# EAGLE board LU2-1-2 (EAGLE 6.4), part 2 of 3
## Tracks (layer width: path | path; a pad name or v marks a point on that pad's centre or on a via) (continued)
N$65 (continued)
  Top 0.305: IC5.13 44.45,78.74 43.18,77.47 43.18,73.66 44.45,72.39 IC4.13 44.45,67.31 43.18,66.04 43.18,62.23 40.64,59.69 40.64,55.88 38.42,53.66 38.42,40.32 37.47,39.37 IC33.15
N$66
  Top 0.305: IC5.11 49.53,78.74 48.26,77.47 48.26,73.66 49.53,72.39 IC4.11 49.53,66.67 48.26,65.41 48.26,56.52 46.35,54.61 41.91,54.61 39.69,52.32 39.69,33.02 38.42,31.75 IC33.12
N$67
  Top 0.305: IC4.8 44.45,77.47 45.72,78.74 45.72,83.19 44.45,84.45 IC5.8
  Route3 0.305: IC33.9 43.81,31.75 45.09,33.02 45.09,53.98 45.72,54.61 45.72,71.75 44.45,73.03 IC4.8
N$68
  Top 0.305: IC4.6 39.37,77.47 40.64,78.74 40.64,83.19 39.37,84.45 IC5.6
  Route3 0.305: IC33.6 44.45,40.64 44.45,53.98 43.18,55.24 43.18,69.22 39.37,73.03 IC4.6
N$69
  Top 0.305: IC4.4 34.29,77.47 35.56,78.74 35.56,83.19 34.29,84.45 IC5.4
  Route3 0.305: IC4.4 34.29,72.39 35.56,71.12 35.56,62.23 38.1,59.69 38.1,45.09 41.27,41.91 IC33.5
N$70
  Top 0.305: IC4.2 29.21,77.47 30.48,78.74 30.48,84.45 29.21,85.72 IC5.2
  Route3 0.305: IC4.2 31.11,78.11 34.92,78.11 35.56,77.47 35.56,73.66 38.1,71.12 38.1,62.23 40.64,59.69 40.64,50.16 41.27,49.53 IC33.2
N$71  (via drill 0.6)
  Top 0.305: JP8.4 96.52,41.91 94.61,43.81 94.61,72.07 v94.3,72.39
  Route2 0.305: v94.3,72.39 118.75,72.39 120.65,70.48 IC7.12
  Bottom 0.305: JP7.4 JP8.4
N$75
  Top 0.305: LED14.K R26.2
N$77  (via drill 0.6)
  Top 0.305: JP8.5 96.52,44.45 95.25,45.72 95.25,73.03 v94.61,73.66
  Bottom 0.305: JP8.5 JP7.5 | IC7.9 120.65,74.3 119.38,73.03 95.89,73.03 95.25,73.66 v94.61,73.66
N$78
  Top 0.305: SV1.6 180.97,45.09 180.97,38.73 180.34,38.1 IC35.7
  Bottom 0.305: SV1.6 RN9.4 | IC20.13 162.56,35.56 163.83,36.83 175.26,36.83 176.53,38.1 IC35.7
N$79  (via drill 0.6)
  Top 0.305: JP8.6 96.52,46.99 95.89,47.62 95.89,74.3 94.93,75.25 v94.3,75.25
  Bottom 0.305: JP7.6 JP8.6 | IC7.7 115.57,74.3 114.94,73.66 96.52,73.66 94.93,75.25 v94.3,75.25
N$84  (via drill 0.6)
  Top 0.305: JP8.7 96.52,50.8 96.52,74.93 v95.25,76.2
  Bottom 0.305: JP8.7 JP7.7 | IC7.5 110.49,74.93 109.86,74.3 97.16,74.3 v95.25,76.2
N$85  (via drill 0.6)
  Top 0.305: JP8.8 97.79,53.34 97.16,53.98 97.16,75.88 v96.84,76.2
  Bottom 0.305: JP7.8 JP8.8 | IC7.3 105.41,75.56 104.78,74.93 98.11,74.93 v96.84,76.2
N$86
  Top 0.305: U6.A0 99.06,22.23 97.79,23.5 97.79,24.77 98.42,25.4 102.87,25.4 104.46,26.99 104.46,46.67 104.14,46.99 IC8.18
N$87
  Top 0.305: U6.A1 96.52,22.23 95.25,23.5 95.25,25.4 95.89,26.04 102.23,26.04 103.82,27.62 103.82,41.59 103.5,41.91 IC8.16
N$88
  Top 0.305: U6.A2 93.98,22.23 92.71,23.5 92.71,25.4 93.98,26.67 101.6,26.67 103.19,28.26 103.19,36.51 102.87,36.83 IC8.14
N$89
  Top 0.305: U6.A3 91.44,22.23 90.17,23.5 90.17,25.4 92.08,27.3 99.06,27.3 100.33,28.57 100.33,30.48 IC8.12
N$90
  Top 0.305: RN5.9 107.95,121.28 109.22,120.02 109.22,116.84 U9.K0
N$91
  Top 0.305: RN5.8 105.41,121.28 106.68,120.02 106.68,117.47 105.41,116.2 U9.K1
N$92
  Route2 0.305: IC8.9 106.68,31.75 102.87,27.94 92.08,27.94 90.17,26.04 90.17,22.86 88.9,21.59 U6.A4
N$93  (via drill 0.6)
  Top 0.305: IC8.7 108.58,36.83 107.95,36.2 107.95,25.4 107.95,24.77 107.95,20.95 v107.31,20.32
  Bottom 0.305: U6.A5 87.63,21.59 100.33,21.59 101.6,20.32 v107.31,20.32
N$94  (via drill 0.6)
  Top 0.305: IC8.5 108.58,41.91 107.31,40.64 107.31,22.86 v106.68,22.23
  Bottom 0.305: U6.A6 83.82,20.95 85.09,22.23 v106.68,22.23
N$95  (via drill 0.6)
  Top 0.305: IC8.3 108.58,46.99 107.63,46.04 107.63,43.5 106.68,42.55 106.68,24.13 v106.05,23.5
  Bottom 0.305: U6.A7 81.28,22.23 81.92,22.86 105.41,22.86 v106.05,23.5
N$96
  Top 0.305: RN15.2 99.06,23.5 100.33,22.23 100.33,19.68 99.06,18.41 U6.K0
N$97
  Top 0.305: RN15.3 96.52,23.5 97.79,22.23 97.79,19.68 96.52,18.41 U6.K1
N$98
  Top 0.305: RN15.4 93.98,23.5 95.25,22.23 95.25,19.68 93.98,18.41 U6.K2
N$99
  Top 0.305: RN15.5 91.44,23.5 92.71,22.23 92.71,19.68 91.44,18.41 U6.K3
N$100
  Top 0.305: RN15.6 88.9,23.5 90.17,22.23 90.17,19.68 88.9,18.41 U6.K4
N$101
  Top 0.305: RN5.7 102.87,121.28 104.14,120.02 104.14,117.47 102.87,116.2 U9.K2
N$102  (via drill 0.6)
  Top 0.305: v160.02,113.03 160.02,93.98 v158.75,92.71
  Route2 0.305: IC26.2 64.77,88.9 66.04,90.17 95.89,90.17 97.79,92.08 158.12,92.08 v158.75,92.71
  Route3 0.305: IC26.2 64.77,86.36 63.5,85.09 63.5,27.3 62.23,26.04 62.23,10.16 60.96,8.89 60.96,5.08 59.69,3.81 54.61,3.81 SW11.2
  Bottom 0.305: IC24.2 184.15,114.94 183.51,114.3 161.29,114.3 v160.02,113.03
N$103
  Top 0.305: R25.2 LED13.K
N$104
  Top 0.305: LED12.K R24.2
N$105
  Top 0.305: RN15.7 86.36,23.5 87.63,22.23 87.63,19.68 86.36,18.41 U6.K5
N$106
  Top 0.305: U6.K6 83.82,18.41 85.09,19.68 85.09,22.23 83.82,23.5 RN15.8
N$107
  Top 0.305: RN15.9 81.28,23.5 82.55,22.23 82.55,19.68 81.28,18.41 U6.K7
N$108  (via drill 0.6)
  Top 0.305: v106.68,44.45 106.68,50.16 102.87,53.98 IC6.19 102.87,59.05 106.68,62.87 106.68,66.04 107.95,67.31 IC7.17
  Bottom 0.305: v106.68,44.45 IC8.17
N$109  (via drill 0.6)
  Top 0.305: IC7.15 113.03,66.67 111.76,65.41 111.76,61.59 110.49,60.33 IC6.16 110.49,55.88 111.12,55.24 111.12,41.27 v110.49,40.64
  Bottom 0.305: v110.49,40.64 106.05,40.64 104.78,39.37 IC8.15
N$110  (via drill 0.6)
  Top 0.305: IC7.13 118.11,67.31 116.84,66.04 116.84,63.5 113.03,59.69 IC6.15 113.03,55.88 114.3,54.61 114.3,38.73 113.67,38.1 112.39,38.1 111.76,37.47 111.76,36.83 v110.49,35.56
  Bottom 0.305: v110.49,35.56 106.68,35.56 105.41,34.29 IC8.13
N$111  (via drill 0.6)
  Top 0.305: IC7.11 123.19,67.31 121.92,66.04 121.92,61.59 120.65,60.33 IC6.12 120.65,55.88 118.11,53.34 118.11,36.2 117.47,35.56 v117.47,31.11
  Bottom 0.305: IC8.11 102.87,29.21 104.14,30.48 116.84,30.48 v117.47,31.11
N$112
  Top 0.305: IC7.8 118.11,73.03 119.38,71.75 119.38,67.31 120.65,66.04 IC6.9 120.65,61.59 119.38,60.33 119.38,55.88 117.47,53.98 117.47,36.83 116.2,35.56 112.39,35.56 111.12,34.29 IC8.8
N$113
  Top 0.305: IC7.6 113.03,73.03 114.3,71.75 114.3,66.67 113.03,65.41 IC6.6 113.03,61.59 111.76,60.33 111.76,40.01 111.12,39.37 IC8.6
N$114
  Top 0.305: IC7.4 107.95,74.3 111.76,70.48 111.76,67.31 110.49,66.04 IC6.5 110.49,61.59 109.22,60.33 109.22,55.88 110.49,54.61 110.49,45.72 IC8.4
N$115
  Top 0.305: IC6.2 102.87,66.04 104.14,67.31 104.14,69.85 | 104.14,69.85 104.14,71.75 102.87,73.03 IC7.2 | IC8.2 108.58,49.53 106.68,51.44 106.68,60.33 109.22,62.87 109.22,69.22 108.58,69.85 104.14,69.85
N$116  (via drill 0.6)
  Top 0.305: JP6.1 88.27,34.29 86.36,36.2 86.36,55.88 87,56.52 87,62.23 v87.63,62.87
  Bottom 0.305: RN22.2 JP5.1 JP6.1 | v87.63,62.87 89.53,62.87 90.17,63.5 104.78,63.5 105.41,64.14 IC6.3
N$117
  Top 0.305: LED11.K R23.2
N$118  (via drill 0.6)
  Top 0.305: IC24.12 201.93,104.78 202.56,104.14 202.56,84.45 208.91,78.11 208.91,44.13 210.19,42.86 210.19,16.51 208.28,14.61 v208.28,9.84
  Route2 0.305: LED14.A 144.78,11.43 151.76,11.43 152.4,12.06 157.48,12.06 158.12,11.43 165.74,11.43 166.37,12.06 202.56,12.06 205.1,9.53 207.96,9.53 v208.28,9.84
N$119  (via drill 0.6)
  Top 0.305: IC24.14 198.75,106.05 198.75,85.72 207.65,76.83 207.65,42.23 208.91,40.96 208.91,17.78 207.01,15.88 207.01,12.06 v206.38,11.43
  Route2 0.305: LED13.A 114.3,13.97 168.91,13.97 169.54,13.34 203.2,13.34 205.1,11.43 v206.38,11.43
N$120  (via drill 0.6)
  Top 0.305: JP6.2 88.27,36.83 87,38.1 87,53.34 87.63,53.98 89.53,53.98 90.81,55.24 90.81,59.69 90.17,60.33 v90.17,61.59
  Bottom 0.305: RN22.3 JP5.2 JP6.2 | v90.17,61.59 90.17,62.23 90.81,62.87 107.31,62.87 107.95,63.5 IC6.4
N$121  (via drill 0.6)
  Top 0.305: IC24.16 195.58,104.14 195.58,87.63 207.01,76.2 207.01,41.27 208.28,40.01 208.28,18.41 205.74,15.88 v205.74,13.97
  Route2 0.305: LED12.A 85.09,15.24 169.54,15.24 170.18,14.61 205.1,14.61 v205.74,13.97
N$122  (via drill 0.6)
  Top 0.305: JP6.3 87.63,40.64 87.63,52.7 88.27,53.34 90.17,53.34 91.44,54.61 v91.44,60.96
  Bottom 0.305: RN22.4 JP5.3 JP6.3 | v91.44,60.96 92.08,61.59 113.03,61.59 115.57,64.14 IC6.7
N$123  (via drill 0.6)
  Top 0.305: v116.2,53.98 116.84,54.61 116.84,60.33 118.11,61.59 IC6.8
  Bottom 0.305: RN22.5 JP5.4 JP6.4 89.53,41.91 90.81,43.18 99.06,43.18 100.33,44.45 100.33,52.7 100.97,53.34 109.86,53.34 110.49,53.98 v116.2,53.98
N$124
  Bottom 0.305: RN22.6 JP5.5 JP6.5 90.17,45.72 98.42,45.72 99.69,46.99 99.69,53.34 100.33,53.98 109.22,53.98 110.49,55.24 117.47,55.24 118.11,55.88 IC6.13
N$125
  Bottom 0.305: RN22.7 JP5.6 JP6.6 90.17,48.26 98.42,48.26 99.06,48.9 99.06,53.98 99.69,54.61 108.58,54.61 109.86,55.88 114.94,55.88 115.57,56.52 IC6.14
N$126
  Bottom 0.305: RN22.8 JP5.7 | 83.19,49.53 JP5.7 | JP5.7 JP6.7 89.53,49.53 90.17,50.16 90.17,53.98 91.44,55.24 107.31,55.24 107.95,55.88 IC6.17
N$127
  Bottom 0.305: RN22.9 JP5.8 JP6.8 88.9,53.98 90.81,55.88 104.78,55.88 105.41,56.52 IC6.18
N$128  (via drill 0.6)
  Route2 0.305: v134.94,70.17 135.25,70.48 141.6,70.48 142.24,69.85 IC10.18
  Route3 0.305: JP12.1 129.54,34.29 130.81,35.56 130.81,52.7 132.72,54.61 132.72,67.94 v134.94,70.17
  Bottom 0.305: JP11.1 JP12.1
N$129  (via drill 0.6)
  Route2 0.305: IC10.16 147.32,69.85 146.05,71.12 133.99,71.12 v133.35,70.48
  Route3 0.305: JP12.2 128.91,36.83 130.18,38.1 130.18,53.02 132.08,54.93 132.08,69.22 v133.35,70.48
  Bottom 0.305: JP11.2 JP12.2
N$130  (via drill 0.6)
  Route2 0.305: IC10.14 152.4,69.85 150.5,71.75 v132.4,71.75
  Route3 0.305: JP12.3 128.91,39.37 129.54,40.01 129.54,53.34 131.44,55.24 131.44,70.8 v132.4,71.75
  Bottom 0.305: JP11.3 JP12.3
N$131  (via drill 0.6)
  Route2 0.305: IC10.12 157.48,69.85 154.31,73.66 v132.72,73.66
  Route3 0.305: JP11.4 123.19,41.91 125.09,43.81 125.09,53.02 125.41,53.34 128.59,53.34 130.81,55.56 130.81,71.75 v132.72,73.66
  Bottom 0.305: JP11.4 JP12.4
N$132  (via drill 0.6)
  Route2 0.305: IC10.9 156.21,74.93 133.35,74.93 v132.72,75.56
  Route3 0.305: JP11.5 123.19,44.45 124.46,45.72 124.46,53.34 125.09,53.98 128.27,53.98 130.18,55.88 130.18,72.71 132.72,75.25 v132.72,75.56
  Bottom 0.305: JP11.5 JP12.5
N$133
  Top 0.305: RN5.6 100.33,121.28 101.6,120.02 101.6,117.47 100.33,116.2 U9.K3
N$134  (via drill 0.6)
  Route2 0.305: v130.49,78.11 131.13,78.74 151.13,78.74 152.4,77.47 IC10.7
  Route3 0.305: JP11.6 123.83,48.9 123.83,53.98 124.46,54.61 127.95,54.61 129.54,56.2 129.54,73.03 131.44,74.93 131.44,77.15 v130.49,78.11
  Bottom 0.305: JP11.6 JP12.6
N$135  (via drill 0.6)
  Route2 0.305: IC10.5 147.32,76.83 146.05,78.11 132.08,78.11 v130.49,76.52
  Route3 0.305: JP11.7 123.19,50.8 123.19,54.29 124.14,55.24 127.64,55.24 128.91,56.52 128.91,73.34 130.49,74.93 v130.49,76.52
  Bottom 0.305: JP11.7 JP12.7
N$136  (via drill 0.6)
  Top 0.305: v165.74,19.68 165.74,27.94 166.37,28.57 167.64,28.57 170.18,31.11 170.18,48.9 170.81,49.53 172.09,49.53 172.72,50.16 172.72,55.24 172.09,55.88 172.09,102.23 171.45,102.87 171.45,105.41 172.09,106.05 v172.09,107.95
  Route2 0.305: LED11.A 53.98,12.7 57.78,16.51 164.47,16.51 165.74,17.78 v165.74,19.68
  Bottom 0.305: IC24.18 185.42,109.22 183.51,109.22 182.88,108.58 182.88,107.31 182.25,106.68 175.26,106.68 173.99,107.95 v172.09,107.95
N$137
  Route3 0.305: LED15.K 77.47,117.47 79.38,119.38 R27.2
N$138  (via drill 0.6)
  Top 0.305: LED16.K 77.47,111.76 78.74,113.03 v78.74,116.84
  Route3 0.305: v78.74,116.84 80.01,118.11 83.82,118.11 R28.2
N$139  (via drill 0.6)
  Route2 0.305: IC10.3 140.97,77.47 133.03,77.47 131.13,75.56 v129.54,75.56
  Route3 0.305: JP11.8 121.92,53.98 123.83,55.88 127.32,55.88 128.27,56.83 128.27,74.93 128.91,75.56 v129.54,75.56
  Bottom 0.305: JP11.8 JP12.8
N$140
  Top 0.305: IC11.18 135.89,44.45 135.89,34.29 135.25,33.66 135.25,20.32 131.44,16.51 128.91,16.51 128.27,17.14 128.27,18.41 129.54,19.68 U7.A0
N$141
  Top 0.305: IC11.16 136.53,40.01 136.53,33.66 135.89,33.02 135.89,19.68 132.08,15.88 126.36,15.88 125.73,16.51 125.73,18.41 127,19.68 U7.A1
N$142
  Top 0.305: IC11.14 137.16,35.56 137.16,33.02 136.53,32.38 136.53,19.05 132.72,15.24 124.46,15.24 123.19,16.51 123.19,18.41 124.46,19.68 U7.A2
N$143
  Top 0.305: IC11.12 137.16,30.48 137.16,18.41 133.35,14.61 122.56,14.61 120.65,16.51 120.65,18.41 121.92,19.68 U7.A3
N$144
  Bottom 0.305: LED17.K R29.2
N$145
  Top 0.305: RN19.12 233.04,102.23 233.04,91.44 235.59,88.9 U16.6
N$146
  Top 0.305: U16.1 229.87,99.69 228.6,100.97 227.97,100.97 225.43,100.97 222.25,104.14 RN19.15
N$147
  Top 0.305: RN19.14 224.79,103.5 226.69,101.6 230.5,101.6 231.14,100.97 231.14,97.79 U16.2
N$148
  Top 0.305: U16.4 231.78,93.34 231.78,101.6 230.5,102.87 228.6,102.87 227.33,104.14 RN19.13
N$149
  Top 0.305: U16.5 228.6,90.17 228.6,99.69 227.97,100.33 224.79,100.33 RN19.16
N$150
  Top 0.305: U16.7 234.95,91.44 234.31,92.08 234.31,103.5 RN19.11
N$151
  Top 0.305: U16.9 236.85,96.52 234.95,98.42 RN19.10
N$152
  Top 0.305: U16.10 RN19.9
N$153  (via drill 0.6)
  Top 0.305: IC17.19 243.84,101.6 245.11,102.87 245.11,116.2 v244.47,116.84
  Bottom 0.305: RN19.5 231.14,114.3 231.14,116.84 231.78,117.47 243.84,117.47 v244.47,116.84
N$154  (via drill 0.6)
  Top 0.305: v251.46,99.69 IC17.16
  Bottom 0.305: RN19.2 222.25,112.39 226.06,108.58 226.06,102.23 227.33,100.97 239.4,100.97 240.66,99.69 v251.46,99.69
N$155  (via drill 0.6)
  Top 0.305: v254.63,100.97 254.63,99.69 254,99.06 IC17.15
  Bottom 0.305: RN19.3 224.79,112.39 231.14,106.05 231.14,102.87 231.78,102.23 240.66,102.23 241.3,101.6 254,101.6 v254.63,100.97
N$156  (via drill 0.6)
  Top 0.305: IC17.12 261.62,97.47 260.35,98.74 260.35,108.58 v259.08,109.86
  Bottom 0.305: RN19.4 228.6,114.3 228.6,116.84 229.87,118.11 245.11,118.11 247.01,116.2 247.01,115.57 250.19,112.39 252.73,112.39 254,111.12 257.81,111.12 v259.08,109.86
N$157  (via drill 0.6)
  Top 0.305: v261.62,99.06 IC17.9
  Bottom 0.305: RN19.1 219.71,108.58 220.98,107.31 220.98,101.6 224.79,97.79 260.35,97.79 v261.62,99.06
N$158
  Bottom 0.305: IC17.6 252.73,102.87 250.82,102.87 250.19,103.5 250.19,105.41 249.56,106.05 240.66,106.05 235.59,111.12 233.04,111.12 232.41,111.76 RN19.6
N$159
  Bottom 0.305: IC17.5 251.46,105.41 250.19,106.68 241.3,106.68 RN19.7
N$160  (via drill 0.6)
  Top 0.305: v243.84,113.03 IC17.2
  Bottom 0.305: RN19.8 v243.84,113.03
N$161
  Top 0.305: U15.6 224.79,88.9 223.52,90.17 223.52,97.16 219.07,101.6 217.17,101.6 216.53,102.23 216.53,118.75 217.81,120.02 226.69,120.02 RN18.5
N$162
  Top 0.305: U15.1 217.17,99.06 215.9,100.33 215.9,119.38 217.17,120.65 224.79,120.65 RN18.4
N$163
  Top 0.305: U15.2 216.53,96.52 215.26,97.79 215.26,119.7 216.85,121.28 222.88,121.28 RN18.3
N$164
  Top 0.305: U15.4 215.9,91.44 214.63,92.71 214.63,120.02 216.53,121.92 220.98,121.92 RN18.2
N$165
  Top 0.305: U15.5 216.53,88.9 214,91.44 214,120.65 216.53,123.19 RN18.1
N$166
  Top 0.305: U15.7 224.79,91.44 224.16,92.08 224.16,97.47 219.39,102.23 217.81,102.23 217.17,102.87 217.17,118.11 218.44,119.38 228.6,119.38 RN18.6
N$167
  Top 0.305: U15.9 226.06,96.52 219.71,102.87 218.12,102.87 217.81,103.19 217.81,117.47 219.07,118.75 230.5,118.75 RN18.7
N$168
  Top 0.305: U15.10 224.79,99.06 220.34,103.5 219.07,103.5 218.44,104.14 218.44,116.84 219.71,118.11 232.41,118.11 RN18.8
N$169  (via drill 0.6)
  Top 0.305: IC16.2 243.84,93.34 242.57,94.61 v242.57,115.57
  Bottom 0.305: v242.57,115.57 RN18.9
N$170  (via drill 0.6)
  Top 0.305: v248.28,112.39 250.19,110.49 250.19,95.89 251.46,94.61 IC16.5
  Bottom 0.305: RN18.10 234.95,116.2 235.59,116.84 242.89,116.84 244.16,115.57 245.11,115.57 v248.28,112.39
N$171  (via drill 0.6)
  Top 0.305: IC16.6 254,94.61 252.73,95.89 252.73,110.49 v251.78,111.44
  Bottom 0.305: v251.78,111.44 251.46,111.12 247.65,111.12 244.47,114.3 233.68,114.3 RN18.11
N$172  (via drill 0.6)
  Top 0.305: v259.08,99.06 260.35,97.79 260.35,95.89 261.62,94.61 IC16.9
  Bottom 0.305: RN18.16 220.98,114.3 220.98,108.58 223.52,106.05 223.52,101.6 224.79,100.33 238.76,100.33 240.66,98.42 258.44,98.42 v259.08,99.06
N$173  (via drill 0.6)
  Top 0.305: v262.89,101.6 262.89,89.53 261.62,88.27 IC16.12
  Bottom 0.305: RN18.15 223.52,114.3 223.52,112.39 228.6,107.31 228.6,102.23 229.24,101.6 240.03,101.6 240.66,100.97 252.73,100.97 254,99.69 257.81,99.69 259.71,101.6 v262.89,101.6
N$174  (via drill 0.6)
  Top 0.305: RN18.14 226.06,114.3 226.06,109.86 228.6,107.31 228.6,104.14 229.24,103.5 230.82,103.5 232.41,101.92 v232.41,82.55
  Bottom 0.305: v232.41,82.55 240.03,82.55 240.66,83.19 243.84,83.19 244.47,83.82 253.37,83.82 254,84.45 IC16.15
N$175  (via drill 0.6)
  Route3 0.305: v248.28,116.84 248.28,114.94 247.01,113.67 247.01,111.76 247.65,111.12 247.65,90.81 251.46,87 IC16.16
  Bottom 0.305: RN18.13 227.33,116.84 229.24,118.75 246.38,118.75 v248.28,116.84
N$176  (via drill 0.6)
  Top 0.305: v239.4,83.82 239.4,89.53 238.76,90.17 235.27,90.17 233.68,91.76 233.68,102.55 231.14,105.09 231.14,114.3 RN18.12
  Bottom 0.305: IC16.19 242.57,83.82 v239.4,83.82
N$177
  Top 0.305: U14.6 237.49,17.14 238.12,16.51 238.12,10.79 239.4,9.53 250.19,9.53 252.73,6.99 RN17.11
N$178
  Top 0.305: U14.1 230.5,27.94 233.68,24.77 233.68,18.73 236.85,15.56 236.85,9.53 238.12,8.26 246.38,8.26 247.65,6.99 RN17.13
N$179
  Top 0.305: RN17.14 245.11,6.99 244.47,7.62 237.49,7.62 236.22,8.89 236.22,15.24 232.41,19.05 232.41,22.86 U14.2
N$180
  Top 0.305: RN17.15 242.57,6.35 241.94,6.99 236.85,6.99 235.59,8.26 235.59,14.61 U14.4
N$181
  Top 0.305: U14.5 230.5,17.78 234.95,13.34 234.95,7.62 237.49,5.08 RN17.16
N$182
  Top 0.305: RN17.12 250.19,6.99 248.28,8.89 238.76,8.89 237.49,10.16 237.49,15.88 235.59,17.78 235.59,19.68 236.22,20.32 U14.7
N$183
  Top 0.305: RN17.10 255.27,6.99 252.09,10.16 240.03,10.16 238.76,11.43 238.76,24.13 U14.9
N$184
  Top 0.305: U14.10 239.4,26.04 239.4,15.24 241.3,13.34 241.3,12.06 242.57,10.79 254,10.79 257.81,6.99 RN17.9
N$185
  Bottom 0.305: RN17.6 252.73,12.06 251.46,10.79 244.47,10.79 243.84,11.43 243.84,13.97 245.11,15.24 IC15.19
N$186
  Bottom 0.305: RN17.4 247.65,13.97 248.28,14.61 252.09,14.61 252.73,15.24 IC15.16
N$187
  Bottom 0.305: RN17.3 246.38,11.43 250.82,11.43 251.46,12.06 251.46,13.34 252.09,13.97 254,13.97 255.27,15.24 IC15.15
N$188
  Bottom 0.305: IC15.12 262.89,17.14 262.25,17.78 244.47,17.78 243.84,17.14 243.84,15.24 242.57,13.97 RN17.2
N$189
  Bottom 0.305: RN17.1 240.03,12.06 241.94,10.16 266.06,10.16 271.14,15.24 271.14,24.77 270.51,25.4 263.52,25.4 262.89,24.77 IC15.9
N$190
  Top 0.305: IC15.6 255.27,20.95 254,19.68 254,14.61 253.37,13.97 251.46,13.97 RN17.5
N$191
  Top 0.305: RN17.7 255.27,13.97 256.54,15.24 256.54,25.4 255.91,26.04 253.37,26.04 252.73,25.4 IC15.5
N$192
  Top 0.305: RN17.8 257.81,12.06 257.18,11.43 244.47,11.43 243.84,12.06 243.84,19.68 245.11,20.95 IC15.2
N$193
  Top 0.305: IC11.9 144.78,31.75 143.51,30.48 143.51,27.94 137.79,22.23 137.79,17.78 133.99,13.97 119.38,13.97 118.11,15.24 118.11,18.41 119.38,19.68 U7.A4
N$194  (via drill 0.6)
  Top 0.305: IC11.7 143.51,36.83 142.88,36.2 142.88,29.84 v142.24,29.21
  Route2 0.305: v142.24,29.21 139.06,26.04 116.2,26.04 115.57,25.4 115.57,23.5 116.84,22.23 U7.A5
N$195  (via drill 0.6)
  Top 0.305: IC11.5 144.78,41.91 142.24,39.37 142.24,31.75 v140.97,30.48 | 114.3,20.95 U7.A6 114.3,22.23 113.03,23.5 113.03,31.11 v113.35,31.43
  Route2 0.305: v113.35,31.43 114.3,32.38 128.91,32.38 130.81,30.48 v140.97,30.48
N$196  (via drill 0.6)
  Top 0.305: IC11.3 144.78,46.99 143.51,45.72 143.51,42.55 140.97,40.01 v140.97,33.02 | U7.A7 111.76,21.59 110.49,22.86 110.49,27.3 111.76,28.57 v111.76,31.75
  Route2 0.305: v111.76,31.75 113.03,33.02 v140.97,33.02
N$197  (via drill 0.6)
  Route3 0.305: RN16.12 229.87,8.89 229.87,13.97 230.5,14.61 232.41,14.61 233.68,15.88 v233.68,35.56
  Bottom 0.305: IC14.2 245.11,34.92 244.47,34.29 240.66,34.29 239.4,35.56 v233.68,35.56
N$198  (via drill 0.6)
  Route3 0.305: RN16.11 232.41,8.89 232.41,13.34 234.31,15.24 234.31,33.66 v234.95,34.29
  Bottom 0.305: IC14.5 252.73,34.29 252.09,33.66 240.03,33.66 238.76,34.92 235.59,34.92 v234.95,34.29
N$199  (via drill 0.6)
  Route3 0.305: RN16.10 234.95,8.89 234.95,32.38 v236.22,33.66
  Bottom 0.305: IC14.6 255.27,33.66 254.63,33.02 239.4,33.02 238.76,33.66 v236.22,33.66
N$200  (via drill 0.6)
  Route3 0.305: RN16.14 220.98,6.35 224.79,10.16 v224.79,33.02
  Bottom 0.305: IC14.9 262.89,33.02 262.25,32.38 226.69,32.38 226.06,33.02 v224.79,33.02
N$201  (via drill 0.6)
  Route3 0.305: RN16.15 218.44,6.35 222.25,10.16 222.25,29.21 222.88,29.84 v222.88,31.75
  Bottom 0.305: IC14.12 262.89,29.84 261.62,31.11 223.52,31.11 v222.88,31.75
N$202  (via drill 0.6)
  Route3 0.305: RN16.16 215.9,6.35 219.71,10.16 219.71,15.24 220.98,16.51 v220.98,30.48
  Bottom 0.305: IC14.15 255.27,29.21 254,30.48 v220.98,30.48
N$203  (via drill 0.6)
  Route3 0.305: RN16.13 223.52,6.35 227.33,10.16 227.33,13.97 228.6,15.24 231.78,15.24 232.41,15.88 v232.41,27.94
  Bottom 0.305: IC14.16 251.46,26.67 233.68,26.67 v232.41,27.94
N$204  (via drill 0.6)
  Route3 0.305: RN16.9 236.22,7.62 v236.22,29.21
  Bottom 0.305: v236.22,29.21 244.47,29.21 245.11,28.57 IC14.19
N$205
  Top 0.305: RN20.2 129.54,23.5 130.81,22.23 130.81,19.05 U7.K0
N$206
  Top 0.305: RN20.3 127,23.5 128.27,22.23 128.27,19.68 127,18.41 U7.K1
N$207
  Top 0.305: RN20.4 124.46,23.5 125.73,22.23 125.73,19.68 124.46,18.41 U7.K2
N$208
  Top 0.305: RN20.5 121.92,23.5 123.19,22.23 123.19,19.68 121.92,18.41 U7.K3
N$209
  Top 0.305: RN20.6 119.38,23.5 120.65,22.23 120.65,19.68 119.38,18.41 U7.K4
N$210
  Top 0.305: RN20.7 116.84,23.5 118.11,22.23 118.11,19.68 116.84,18.41 U7.K5
N$211
  Top 0.305: RN20.8 114.3,23.5 115.57,22.23 115.57,19.68 114.3,18.41 U7.K6
N$212
  Top 0.305: RN20.9 111.76,23.5 113.03,22.23 113.03,19.68 111.76,18.41 U7.K7
N$213
  Top 0.305: U13.10 225.43,27.94 224.16,26.67 224.16,15.24 226.06,13.34 RN16.5
N$214
  Top 0.305: U13.9 226.69,25.4 224.79,23.5 224.79,16.51 RN16.6
N$215
  Top 0.305: U13.7 226.69,20.32 226.06,19.68 226.06,17.14 227.97,15.24 228.6,15.24 RN16.7
N$216
  Top 0.305: U13.5 219.71,16.51 220.98,15.24 RN16.3
N$217
  Top 0.305: U13.4 219.07,20.32 218.44,19.68 RN16.2
N$218
  Top 0.305: U13.2 218.44,25.4 215.9,22.86 RN16.1
N$219
  Top 0.305: U13.1 220.98,27.94 223.52,25.4 RN16.4
N$220
  Top 0.305: U13.6 229.24,15.88 230.5,15.88 RN16.8
N$221  (via drill 0.6)
  Top 0.305: IC11.17 139.7,45.72 IC9.19 139.7,60.33 138.43,61.59 v138.43,67.31
  Bottom 0.305: v138.43,67.31 143.51,67.31 IC10.17
N$222  (via drill 0.6)
  Top 0.305: IC10.15 149.86,67.31 148.59,66.04 148.59,60.33 147.32,59.05 IC9.16 147.32,55.88 147.96,55.24 147.96,41.27 v147.32,40.64
  Bottom 0.305: v147.32,40.64 142.24,40.64 140.97,39.37 IC11.15
N$223  (via drill 0.6)
  Top 0.305: IC11.13 139.7,35.56 139.7,43.81 140.97,45.09 v140.97,51.44 | IC10.13 153.67,67.31 153.67,62.87 149.86,59.05 IC9.15
  Bottom 0.305: v140.97,51.44 141.6,51.44 144.78,54.61 147.32,54.61 IC9.15
N$224  (via drill 0.6)
  Top 0.305: IC10.11 160.02,67.31 158.75,66.04 158.75,60.33 157.48,59.05 IC9.12 | v141.6,42.55 140.34,41.27 140.34,34.29 139.7,33.66 139.7,29.84 139.06,29.21 IC11.11
  Bottom 0.305: IC9.12 157.48,56.52 154.94,53.98 150.5,53.98 149.86,53.34 149.86,45.72 147.32,43.18 142.24,43.18 v141.6,42.55
N$225
  Top 0.305: IC10.8 154.94,73.66 156.21,72.39 156.21,67.31 157.48,66.04 IC9.9 151.13,58.42 151.13,55.88 149.22,53.98 149.22,36.83 146.69,34.29 IC11.8
N$226
  Top 0.305: IC10.6 149.86,73.66 151.13,72.39 151.13,67.31 149.86,66.04 IC9.6 149.86,60.33 148.59,59.05 148.59,40.01 147.96,39.37 IC11.6
N$227
  Top 0.305: IC10.4 144.78,73.66 146.05,72.39 146.05,67.31 147.32,66.04 IC9.5 147.32,61.59 146.05,60.33 146.05,55.88 147.32,54.61 147.32,45.72 IC11.4
N$228
  Top 0.305: IC10.2 139.7,73.03 140.97,71.75 140.97,67.94 139.7,66.67 IC9.2 139.7,61.59 140.97,60.33 140.97,53.34 144.78,49.53 IC11.2
N$229  (via drill 0.6)
  Top 0.305: RN12.2 133.99,34.29 135.25,35.56 135.25,55.88 135.89,56.52 135.89,62.87 135.25,63.5 134.3,63.5 v133.99,63.18
  Route2 0.305: v133.99,63.18 141.29,63.18 142.24,64.14 IC9.3
  Bottom 0.305: JP9.1 JP10.1 120.02,34.29 121.28,35.56 130.18,35.56 131.44,34.29 RN12.2
N$230
  Top 0.305: IC35.9 181.61,35.56 181.61,43.18 SV1.5
  Bottom 0.305: SV1.5 RN9.5 | IC35.9 175.26,33.02 173.99,31.75 164.47,31.75 163.19,30.48 IC20.11
N$231  (via drill 0.6)
  Top 0.305: RN12.3 133.35,36.83 134.62,38.1 134.62,56.2 135.25,56.83 135.25,61.28 v134.62,61.91
  Route2 0.305: IC9.4 144.78,64.14 142.56,61.91 v134.62,61.91
  Bottom 0.305: JP9.2 JP10.2 120.02,36.83 121.28,38.1 130.18,38.1 131.44,36.83 RN12.3
N$232  (via drill 0.6)
  Top 0.305: RN12.4 132.72,39.37 133.99,40.64 133.99,56.52 134.62,57.15 134.62,59.69 v133.99,60.33
  Route2 0.305: v133.99,60.33 147.96,60.33 IC9.7
  Bottom 0.305: JP9.3 JP10.3 120.02,39.37 121.28,40.64 130.18,40.64 131.44,39.37 RN12.4
N$233  (via drill 0.6)
  Top 0.305: RN12.5 133.35,43.18 133.35,58.42 v133.67,58.74
  Route2 0.305: v133.67,58.74 148.91,58.74 IC9.8
  Bottom 0.305: JP9.4 JP10.4 120.02,41.91 121.28,43.18 130.18,43.18 131.44,41.91 RN12.5
N$234
  Bottom 0.305: JP9.5 JP10.5 120.02,44.45 121.28,45.72 130.18,45.72 131.44,44.45 RN12.6 135.89,44.45 137.16,45.72 147.32,45.72 148.59,46.99 148.59,53.66 149.54,54.61 153.03,54.61 154.94,56.52 IC9.13
N$235
  Bottom 0.305: JP9.6 JP10.6 120.65,48.26 130.18,48.26 131.44,46.99 RN12.7 135.25,46.99 136.53,48.26 146.69,48.26 147.96,49.53 147.96,53.98 149.22,55.24 150.5,55.24 IC9.14
N$236
  Bottom 0.305: JP9.7 JP10.7 120.65,50.8 130.18,50.8 131.44,49.53 RN12.8 133.35,49.53 138.43,54.61 140.97,54.61 141.6,55.24 143.51,55.24 144.78,56.52 IC9.17
N$237
  Bottom 0.305: JP9.8 JP10.8 120.65,53.34 130.18,53.34 131.44,52.07 RN12.9 134.62,52.07 137.79,55.24 140.34,55.24 IC9.18
N$238
  Bottom 0.305: R30.2 73.66,100.33 75.56,100.33 76.83,99.06 LED18.K
N$239
  Route3 0.305: IC18.18 176.53,19.68 175.26,20.95 161.29,20.95 160.66,21.59 152.4,21.59 151.13,22.86 151.13,29.21 152.4,30.48 JP13.1
  Bottom 0.305: JP13.1 JP14.1
N$240
  Route3 0.305: IC18.16 181.61,20.32 180.34,21.59 161.93,21.59 161.29,22.23 154.31,22.23 153.67,22.86 153.67,35.56 JP13.2
  Bottom 0.305: JP13.2 JP14.2
N$241
  Route3 0.305: IC18.14 186.69,20.95 185.42,22.23 162.56,22.23 161.93,22.86 156.84,22.86 156.21,23.5 156.21,38.73 155.57,39.37 JP14.3
  Bottom 0.305: JP13.3 JP14.3
N$242
  Route3 0.305: IC18.12 191.77,21.59 190.5,22.86 165.74,22.86 163.19,25.4 158.75,25.4 157.48,26.67 157.48,40.64 156.21,41.91 JP14.4
  Bottom 0.305: JP13.4 JP14.4
N$243
  Route3 0.305: IC18.9 191.77,24.77 190.5,23.5 166.05,23.5 161.93,27.62 161.93,41.27 161.29,41.91 159.38,41.91 156.84,44.45 JP14.5
  Bottom 0.305: JP13.5 JP14.5
N$244
  Route3 0.305: IC18.7 186.69,25.4 185.42,24.13 166.37,24.13 162.56,27.94 162.56,43.81 161.93,44.45 159.38,44.45 156.84,46.99 JP14.6
  Bottom 0.305: JP13.6 JP14.6
N$245
  Route3 0.305: IC18.5 181.61,26.04 180.34,24.77 166.69,24.77 163.19,28.26 163.19,45.72 161.93,46.99 159.38,46.99 156.84,49.53 JP14.7
  Bottom 0.305: JP13.7 JP14.7
N$246
  Route3 0.305: IC18.3 176.53,26.04 175.9,25.4 167,25.4 163.83,28.57 163.83,48.26 162.56,49.53 158.75,49.53 156.21,52.07 JP14.8
  Bottom 0.305: JP13.8 JP14.8
N$247  (via drill 0.6)
  Top 0.305: U8.A0 160.02,19.68 158.75,18.41 158.75,14.61 160.02,13.34 160.02,12.06 160.66,11.43 161.29,11.43 163.19,9.53 v163.19,7.62
  Bottom 0.305: v163.19,7.62 175.26,7.62 IC19.18
N$248  (via drill 0.6)
  Top 0.305: SV1.4 183.51,41.91 184.78,40.64 v184.78,33.02
  Bottom 0.305: SV1.4 RN9.6 | IC20.8 168.91,35.56 IC35.12 173.99,33.02 175.26,34.29 180.34,34.29 181.61,33.02 v184.78,33.02
N$249  (via drill 0.6)
  Top 0.305: U8.A1 157.48,19.68 156.21,18.41 156.21,10.79 v155.57,10.16
  Bottom 0.305: IC19.16 181.61,9.53 179.71,11.43 165.1,11.43 163.83,10.16 v155.57,10.16
N$250  (via drill 0.6)
  Top 0.305: U8.A2 154.94,19.68 153.67,18.41 v153.67,10.16
  Bottom 0.305: IC19.14 186.69,10.79 185.42,12.06 164.47,12.06 163.19,10.79 156.84,10.79 156.21,11.43 154.94,11.43 v153.67,10.16
N$251  (via drill 0.6)
  Top 0.305: U8.A3 152.4,19.68 151.13,18.41 v151.13,12.7
  Bottom 0.305: IC19.12 191.77,11.43 190.5,12.7 163.83,12.7 162.56,11.43 157.48,11.43 156.21,12.7 v151.13,12.7
N$252  (via drill 0.6)
  Top 0.305: U8.A4 149.86,19.68 148.59,18.41 148.59,15.88 149.22,15.24 v149.22,12.7
  Bottom 0.305: v149.22,12.7 150.5,13.97 164.47,13.97 165.1,13.34 190.5,13.34 191.77,14.61 IC19.9
N$253  (via drill 0.6)
  Top 0.305: U8.A5 147.32,19.68 146.05,18.41 146.05,15.88 147.32,14.61 v147.32,12.7
  Bottom 0.305: v147.32,12.7 149.22,14.61 165.1,14.61 165.74,13.97 185.42,13.97 186.69,15.24 IC19.7
N$254  (via drill 0.6)
  Top 0.305: U8.A6 144.78,19.68 143.51,18.41 143.51,16.51 145.41,14.61 v145.41,12.7
  Bottom 0.305: v145.41,12.7 147.96,15.24 165.74,15.24 166.37,14.61 179.71,14.61 IC19.5
N$255
  Top 0.305: RN5.5 97.79,121.28 99.06,120.02 99.06,117.47 97.79,116.2 U9.K4
N$257  (via drill 0.6)
  Top 0.305: U8.A7 140.34,18.41 v140.34,17.78
  Bottom 0.305: v140.34,17.78 142.24,15.88 166.37,15.88 167,15.24 175.26,15.24 IC19.3
N$258
  Top 0.305: RN21.2 160.02,23.5 161.29,22.23 161.29,19.68 160.02,18.41 U8.K0
N$259
  Top 0.305: RN21.3 157.48,23.5 158.75,22.23 158.75,19.68 157.48,18.41 U8.K1
N$260
  Top 0.305: RN21.4 154.94,23.5 156.21,22.23 156.21,19.68 154.94,18.41 U8.K2
N$261
  Top 0.305: RN21.5 152.4,23.5 153.67,22.23 153.67,19.68 152.4,18.41 U8.K3
N$262
  Top 0.305: RN21.6 149.86,23.5 151.13,22.23 151.13,19.68 149.86,18.41 U8.K4
N$263
  Top 0.305: RN21.7 147.32,23.5 148.59,22.23 148.59,19.68 147.32,18.41 U8.K5
N$264
  Top 0.305: RN21.8 144.78,23.5 146.05,22.23 146.05,19.68 144.78,18.41 U8.K6
N$265
  Top 0.305: RN21.9 142.24,23.5 143.51,22.23 143.51,19.68 142.24,18.41 U8.K7
N$266
  Top 0.305: IC19.17 179.07,11.43 177.8,12.7 177.8,17.14 179.07,18.41 IC18.17 179.07,22.23 177.8,23.5 177.8,27.3 180.97,30.48 185.42,30.48 187.96,33.02 187.96,56.52 186.69,57.78 182.25,57.78 181.61,58.42 IC12.19
N$267
  Top 0.305: IC19.15 184.15,11.43 182.88,12.7 182.88,17.14 184.15,18.41 IC18.15 184.15,21.59 182.88,22.86 182.88,27.3 184.78,29.21 186.69,29.21 189.23,31.75 IC12.16
N$268
  Top 0.305: IC19.13 189.23,11.43 187.96,12.7 187.96,17.14 189.23,18.41 IC18.13 189.23,21.59 187.96,22.86 187.96,27.94 190.5,30.48 190.5,57.15 191.77,58.42 191.77,59.05 IC12.15
N$269
  Top 0.305: IC19.11 194.31,11.43 193.04,12.7 193.04,17.14 194.31,18.41 IC18.11 194.31,21.59 193.04,22.86 193.04,50.16 194.94,52.07 197.49,52.07 199.39,53.98 IC12.12
N$270  (via drill 0.6)
  Top 0.305: IC19.8 190.5,17.78 190.5,21.59 189.23,22.86 IC18.8 189.23,27.94 191.13,29.84 191.13,56.52 193.04,58.42 193.04,64.14 v194.31,65.41
  Bottom 0.305: v194.31,65.41 198.75,65.41 199.39,66.04 IC12.9
N$271
  Top 0.305: IC19.6 184.15,17.14 185.42,18.41 185.42,21.59 184.15,22.86 IC18.6 186.06,28.57 187.32,28.57 189.87,31.11 189.87,57.78 190.5,58.42 190.5,63.5 191.77,64.77 IC12.6
N$272
  Top 0.305: IC19.4 180.34,17.78 180.34,22.23 179.07,23.5 IC18.4 182.25,29.84 186.06,29.84 188.59,32.38 188.59,57.78 187.96,58.42 187.96,63.5 189.23,64.77 IC12.5
N$273  (via drill 0.6)
  Top 0.305: IC19.2 173.99,17.14 175.26,18.41 175.26,22.23 173.99,23.5 IC18.2 173.99,27.94 174.62,28.57 v174.62,65.41
  Bottom 0.305: v174.62,65.41 180.97,65.41 181.61,66.04 IC12.2
N$274  (via drill 0.6)
  Top 0.305: RN11.2 45.09,37.47 45.09,46.35 v46.35,47.62
  Bottom 0.305: RN11.2 JP1.1 JP2.1 | v46.35,47.62 45.72,46.99 IC33.3
N$275
  Bottom 0.305: IC24.9 201.93,118.11 201.29,118.75 178.44,118.75 177.16,117.47 151.13,117.47 147.96,114.3 127.64,114.3 127,113.67 81.92,113.67 81.28,114.3 LED15.A
N$276  (via drill 0.6)
  Top 0.305: RN11.3 46.35,38.73 v46.35,44.45
  Bottom 0.305: RN11.3 JP1.2 JP2.2 | v46.35,44.45 IC33.4
N$277
  Bottom 0.305: JP2.3 JP1.3 RN11.4 46.99,39.37 44.45,36.83 IC33.7
N$278
  Bottom 0.305: JP2.4 JP1.4 RN11.5 44.45,38.1 42.55,38.1 41.91,37.47 41.91,35.56 IC33.8
N$279
  Bottom 0.305: JP1.5 RN11.6 44.45,40.64 41.91,40.64 IC33.13 | 52.7,44.45 JP1.5 | JP1.5 JP2.5
N$280
  Bottom 0.305: JP2.6 JP1.6 RN11.7 46.99,45.72 42.55,45.72 40.64,43.81 40.64,40.64 36.83,36.83 IC33.14
N$281
  Bottom 0.305: JP2.7 JP1.7 RN11.8 46.35,49.53 45.09,48.26 41.91,48.26 38.1,44.45 IC33.17
N$282
  Bottom 0.305: JP2.8 JP1.8 RN11.9 46.35,52.07 45.09,50.8 41.27,50.8 37.47,46.99 IC33.18
N$283
  Bottom 0.305: RN9.7 SV1.3 176.53,39.37 175.26,38.1 IC35.14 168.91,40.64 IC20.6
N$284
  Route2 0.305: IC35.16 175.26,43.18 176.53,41.91 176.53,40.01 177.16,39.37 180.34,39.37 180.97,38.73 180.97,37.47 181.61,36.83 SV1.2
  Bottom 0.305: SV1.2 RN9.8 | IC35.16 168.91,45.72 IC20.4
N$285  (via drill 0.6)
  Top 0.305: IC35.18 172.09,48.26 172.72,47.62 v172.72,34.29
  Route2 0.305: v172.72,34.29 SV1.1
  Bottom 0.305: SV1.1 RN9.9 | IC20.2 168.91,50.8 IC35.18
N$287  (via drill 0.6)
  Top 0.305: S2.9 20.32,13.97 21.59,15.24 21.59,21.59 20.32,22.86 RN10.2 20.32,24.77 24.13,27.94 24.13,52.07 22.86,53.34 22.86,56.52 22.54,56.83 v22.54,57.47
  Bottom 0.305: IC21.17 33.02,58.42 23.81,58.42 22.86,57.47 v22.54,57.47
N$288  (via drill 0.6)
  Top 0.305: S2.10 22.86,13.97 24.13,15.24 24.13,21.59 22.86,22.86 RN10.3 22.86,25.4 24.77,27.3 24.77,52.7 23.5,53.98 23.5,58.42 v22.86,59.05
  Bottom 0.305: IC21.15 39.37,57.78 37.47,59.69 23.5,59.69 v22.86,59.05
N$289  (via drill 0.6)
  Top 0.305: S2.11 25.4,13.97 26.67,15.24 26.67,21.59 25.4,22.86 RN10.4 25.4,53.34 24.13,54.61 24.13,59.44 23.11,60.45 v23.11,62.48
  Bottom 0.305: IC21.13 41.27,60.33 23.88,60.33 23.11,61.09 v23.11,62.48
N$290  (via drill 0.6)
  Top 0.305: S2.12 27.94,13.97 29.21,15.24 29.21,21.59 27.94,22.86 RN10.5 27.94,25.4 26.04,27.3 26.04,53.98 24.77,55.24 24.77,60.33 24.13,60.96 v24.13,61.59
  Bottom 0.305: v24.13,61.59 45.09,61.59 IC21.11
N$291  (via drill 0.6)
  Top 0.305: S2.13 30.48,13.97 31.75,15.24 31.75,21.59 30.48,22.86 RN10.6 30.48,25.4 26.67,29.21 26.67,54.61 25.4,55.88 25.4,62.23 v24.13,63.5
  Bottom 0.305: v24.13,63.5 43.81,63.5 44.45,64.14 IC21.8
N$292  (via drill 0.6)
  Top 0.305: S2.14 33.02,13.97 34.29,15.24 34.29,21.59 33.02,22.86 RN10.7 33.02,26.04 31.75,27.3 30.48,27.3 29.21,28.57 29.21,54.61 27.94,55.88 27.94,60.01 26.04,61.91 26.04,63.5 24.77,64.77 v24.77,66.04
  Bottom 0.305: v24.77,66.04 38.1,66.04 IC21.6
N$293
  Top 0.305: S2.15 35.56,13.97 36.83,15.24 36.83,21.59 35.56,22.86 RN10.8 35.56,26.67 33.02,29.21 33.02,59.69 34.29,60.96 IC21.4
N$294
  Top 0.305: RN10.9 38.1,22.86 39.37,21.59 39.37,15.24 38.1,13.97 S2.16
  Route3 0.305: IC21.2 29.21,62.87 33.02,59.05 33.02,29.21 35.56,26.67 37.47,26.67 38.1,26.04 RN10.9
N$295
  Top 0.305: IC27.8 80.01,60.33 78.74,59.05 78.74,55.24 76.83,53.34 76.83,14.61 74.3,12.06 74.3,5.71 72.39,3.81 67.31,3.81 SW13.2
N$296
  Bottom 0.305: LED16.A 83.82,113.03 127.64,113.03 128.27,113.67 148.59,113.67 151.76,116.84 177.8,116.84 179.07,118.11 196.22,118.11 196.85,117.47 IC24.7
N$297  (via drill 0.6)
  Top 0.305: IC27.7 77.47,60.33 76.2,59.05 76.2,16.51 73.03,13.34 v73.03,6.99
  Route2 0.305: SW14.2 96.52,8.26 95.25,9.53 78.74,9.53 76.2,6.99 v73.03,6.99
N$298  (via drill 0.6)
  Top 0.305: IC27.6 74.93,60.33 73.66,59.05 v73.66,26.67
  Route3 0.305: SW15.2 127,11.43 124.46,13.97 77.47,13.97 73.66,17.78 v73.66,26.67
N$299
  Bottom 0.305: IC24.5 191.77,116.84 191.13,117.47 179.71,117.47 178.44,116.2 152.4,116.2 149.22,113.03 128.91,113.03 128.27,112.39 88.27,112.39 LED17.A
N$300
  Bottom 0.305: SW11.1 54.61,3.81 53.34,3.81 52.07,5.08 R22.1
N$301
  Bottom 0.305: SW10.1 85.09,3.81 84.45,3.81 83.19,5.08 R21.1
N$302
  Bottom 0.305: SW8.1 114.3,5.08 R20.1
N$303
  Bottom 0.305: SW6.1 147.32,3.17 145.41,5.08 R19.1
N$304
  Top 0.305: SW5.1 214.63,127 R18.1
N$305
  Top 0.305: SW4.1 227.33,127 R17.1
N$306
  Top 1.422: 5.08,116.84 5.08,116.98
  Top 1.778: D1.C D2.A 8.89,87.63 7.62,88.9 7.62,91.44 3.81,95.25 3.81,115.57 5.08,116.84 | 5.08,116.98 P1.3
N$307
  Top 1.778: C1.+ 15.24,73.66 U1.S 12.7,76.2 11.43,77.47 10.16,77.47 6.35,81.28 6.35,86.36 5.08,87.63 D2.C D3.C
  Route3 1.27: C1.+ 15.88,80.64 15.88,94.61 19.05,97.79 C2.1
  Bottom 1.422: C2.1 19.05,97.79 15.88,94.61 15.88,80.64 C1.+
N$308
  Bottom 0.305: IC24.3 186.69,116.2 186.06,116.84 180.34,116.84 179.07,115.57 153.03,115.57 147.96,110.49 144.78,110.49 143.51,111.76 88.9,111.76 82.55,105.41 82.55,101.6 LED18.A
N$309
  Top 0.305: RN5.4 95.25,121.28 96.52,120.02 96.52,117.47 95.25,116.2 U9.K5
N$310
  Top 0.305: SW3.1 240.03,127 R16.1
N$311
  Top 0.305: SW2.1 252.73,127 R14.1
N$312
  Top 0.305: SW1.1 251.46,115.57 R1.1
N$313
  Top 0.305: SW9.1 189.87,4.45 187.01,4.45 R8.1
N$314
  Bottom 0.305: R31.2 LED19.K
N$315  (via drill 0.6)
  Route2 0.305: LED19.A 89.53,93.98 91.44,95.89 130.81,95.89 131.44,95.25 171.45,95.25 172.72,96.52 196.53,96.52 v197.17,97.16
  Route3 0.305: IC25.18 194.31,48.26 193.04,49.53 193.04,55.88 195.58,58.42 195.58,95.89 196.85,97.16 v197.17,97.16
N$316
  Top 0.305: R32.2 217.17,60.96 LED20.K
N$317  (via drill 0.6)
  Top 0.305: v214.63,45.72 214.63,53.98 215.26,54.61 215.26,62.87 215.9,63.5 218.44,63.5 LED20.A
  Route2 0.305: IC25.16 198.12,43.18 199.39,44.45 213.36,44.45 v214.63,45.72
N$318  (via drill 0.6)
  Top 0.305: v161.29,112.39 160.66,111.76 160.66,93.34 160.02,92.71 v160.02,92.08
  Route2 0.305: IC26.3 69.22,89.53 96.52,89.53 98.42,91.44 159.38,91.44 v160.02,92.08 | SW10.2 82.55,3.81 74.3,3.81 v73.03,2.54
  Route3 0.305: IC26.3 67.31,86.36 68.58,85.09 68.58,27.3 69.85,26.04 69.85,17.78 71.75,15.88 71.75,3.17 72.39,2.54 v73.03,2.54
  Bottom 0.305: IC24.4 189.23,114.94 187.96,113.67 162.56,113.67 v161.29,112.39
N$319
  Top 0.305: RN5.3 92.71,121.28 93.98,120.02 93.98,117.47 92.71,116.2 U9.K6
N$320  (via drill 0.6)
  Top 0.305: v162.56,111.76 161.29,110.49 v161.29,91.44
  Route2 0.305: IC26.4 69.85,88.27 70.48,88.9 97.16,88.9 99.06,90.81 160.66,90.81 v161.29,91.44
  Route3 0.305: IC26.4 69.85,85.09 71.12,83.82 71.12,53.98 69.85,52.7 69.85,27.94 73.03,24.13 73.03,15.88 77.47,11.43 112.39,11.43 114.3,9.53 SW8.2
  Bottom 0.305: IC24.6 194.31,114.94 192.41,113.03 163.83,113.03 v162.56,111.76
N$321  (via drill 0.6)
  Top 0.305: IC24.8 199.39,113.03 200.66,111.76 200.66,104.78 201.93,103.5 201.93,83.82 208.28,77.47 208.28,43.18 209.55,41.91 209.55,17.14 207.65,15.24 207.65,10.79 207.01,10.16 207.01,8.26 208.28,6.99 v208.91,6.99
  Route2 0.305: SW6.2 145.41,2.54 146.69,3.81 162.56,3.81 168.91,10.16 201.61,10.16 204.47,7.3 208.6,7.3 v208.91,6.99
  Route3 0.305: IC26.5 72.39,85.09 73.66,83.82 73.66,34.29 74.93,33.02 74.93,17.78 78.11,14.61 141.6,14.61 142.24,13.97 142.24,8.89 144.78,6.35 SW6.2
N$322
  Top 0.305: RN5.2 90.17,121.28 91.44,120.02 91.44,117.47 90.17,116.2 U9.K7
N$323  (via drill 0.6)
  Top 0.305: U9.A3 100.33,117.47 99.06,116.2 99.06,106.68 97.16,104.78 97.16,84.45 93.34,80.64 v93.34,80.01
  Bottom 0.305: v93.34,80.01 93.34,79.38 95.25,77.47 119.38,77.47 120.65,78.74 IC28.12
N$324  (via drill 0.6)
  Top 0.305: U9.A2 102.87,117.47 101.6,116.2 101.6,107.31 97.79,103.5 97.79,83.19 94.93,80.33 v94.93,80.01
  Bottom 0.305: v94.93,80.01 94.93,79.69 96.52,78.11 114.94,78.11 115.57,78.74 IC28.14
N$325  (via drill 0.6)
  Top 0.305: U9.A1 105.41,117.47 104.14,116.2 104.14,107.95 98.42,102.23 98.42,81.92 v96.52,80.01
  Bottom 0.305: v96.52,80.01 97.79,78.74 109.86,78.74 110.49,79.38 IC28.16
N$326  (via drill 0.6)
  Top 0.305: SW5.2 212.09,124.46 210.19,122.56 v210.19,107 210.19,92.71 v208.28,90.81
  Route2 0.305: IC26.6 74.93,86.36 76.2,85.09 106.05,85.09 106.68,85.72 106.68,88.27 107.31,88.9 172.72,88.9 174.62,90.81 v208.28,90.81
  Bottom 0.305: IC24.11 204.47,107.31 205.1,106.68 208.91,106.68 209.23,107 v210.19,107
N$327  (via drill 0.6)
  Top 0.305: v211.46,106.05 211.46,107.31 210.82,107.95 210.82,121.92 213.36,124.46 217.17,124.46 219.71,127 223.52,127 SW4.2 | 211.46,105.41 v211.46,106.05 | v211.46,106.05 v211.46,92.08
  Route2 0.305: IC26.7 77.47,87 78.74,85.72 103.5,85.72 104.14,86.36 104.14,88.9 104.78,89.53 172.09,89.53 173.99,91.44 205.74,91.44 206.38,92.08 v211.46,92.08
  Bottom 0.305: IC24.13 199.39,106.68 200.03,106.05 208.91,106.05 209.55,105.41 210.82,105.41 v211.46,106.05
N$328  (via drill 0.6)
  Top 0.305: IC24.15 198.12,104.14 198.12,93.98 v196.85,92.71
  Route2 0.305: IC26.8 80.01,87 80.64,86.36 100.97,86.36 101.6,87 101.6,88.27 103.5,90.17 171.45,90.17 173.35,92.08 196.22,92.08 v196.85,92.71
  Bottom 0.305: SW3.2 237.49,125.73 236.22,124.46 236.22,122.56 235.59,121.92 218.44,121.92 206.38,109.86 194.94,109.86 194.31,109.22 IC24.15
N$329  (via drill 0.6)
  Top 0.305: IC24.17 190.5,106.68 190.5,94.61 v189.23,93.34 | IC26.9 82.55,88.9 85.09,91.44 v85.72,91.44
  Route2 0.305: v85.72,91.44 86.36,90.81 95.25,90.81 97.16,92.71 156.84,92.71 158.75,94.61 172.09,94.61 172.72,93.98 188.59,93.98 v189.23,93.34
  Bottom 0.305: SW2.2 250.19,127 244.47,121.28 219.07,121.28 207.01,109.22 196.22,109.22 195.58,108.58 195.58,107.31 194.94,106.68 189.87,106.68 189.23,107.31 IC24.17
N$330  (via drill 0.6)
  Top 0.305: v200.66,71.12 200.66,51.44 201.29,50.8 IC25.2 | v211.77,112.39 211.77,111.44 211.46,111.12 211.46,108.58 212.72,107.31 v212.72,71.12
  Bottom 0.305: IC27.2 64.77,66.04 65.41,66.67 136.53,66.67 137.16,66.04 140.97,66.04 141.6,66.67 170.18,66.67 174.62,71.12 v200.66,71.12 v212.72,71.12 | SW1.2 251.46,118.11 248.92,120.65 219.71,120.65 211.77,112.71 v211.77,112.39
N$331  (via drill 0.6)
  Top 0.305: IC27.3 67.31,60.33 66.04,59.05 66.04,54.61 66.67,53.98 67.94,53.98 68.58,53.34 68.58,41.91 v71.12,39.37 | IC25.4 202.56,45.72 201.93,45.09 201.93,15.88 203.2,14.61 v203.2,5.08
  Route2 0.305: v203.2,5.08 201.93,5.08 200.66,3.81 190.5,3.81 SW9.2
  Route3 0.305: SW9.2 187.96,3.81 187.96,6.35 186.69,7.62 169.54,7.62 166.37,10.79 166.37,13.34 163.83,15.88 79.38,15.88 76.2,19.05 76.2,38.1 v74.93,39.37
  Bottom 0.305: v71.12,39.37 v74.93,39.37
N$332  (via drill 0.6)
  Top 0.305: IC27.5 72.39,60.33 71.12,59.05 71.12,48.9 72.39,47.62 v72.39,36.83
  Route3 0.305: SW16.2 157.48,13.97 156.21,15.24 78.74,15.24 75.56,18.41 75.56,36.2 v74.93,36.83
  Bottom 0.305: v72.39,36.83 v74.93,36.83
N$333  (via drill 0.6)
  Top 0.305: IC27.4 69.85,60.33 68.58,59.05 68.58,54.29 69.22,53.66 69.22,43.5 v71.44,41.27
  Route3 0.305: v74.93,41.27 76.83,39.37 76.83,19.68 80.01,16.51 164.47,16.51 166.37,14.61 197.49,14.61 201.29,10.79 201.29,5.4 203.2,3.49 SW17.2
  Bottom 0.305: v74.93,41.27 v71.44,41.27
N$334
  Top 0.305: U9.A0 107.95,117.47 106.68,116.2 106.68,108.58 101.6,103.5 101.6,87 105.41,83.19 IC28.18
N$335  (via drill 0.6)
  Top 0.305: U9.A4 97.79,117.47 96.52,116.2 96.52,106.05 95.89,105.41 v95.89,93.98
  Bottom 0.305: IC28.9 120.65,90.17 120.02,90.81 99.06,90.81 v95.89,93.98
N$336  (via drill 0.6)
  Top 0.305: U9.A5 95.25,117.47 93.98,116.2 93.98,94.3 v94.3,93.98
  Bottom 0.305: IC28.7 115.57,88.9 114.3,90.17 98.42,90.17 96.52,92.08 96.2,92.08 v94.3,93.98
N$337  (via drill 0.6)
  Top 0.305: U9.A6 92.71,117.47 91.44,116.2 91.44,113.67 92.71,112.39 92.71,93.98 v94.61,92.08
  Bottom 0.305: IC28.5 110.49,88.27 109.22,89.53 97.47,89.53 94.93,92.08 v94.61,92.08
N$338  (via drill 0.6)
  Top 0.305: U9.A7 90.17,117.47 88.9,116.2 88.9,114.3 92.08,111.12 92.08,92.71 v92.71,92.08
  Bottom 0.305: IC28.3 105.41,88.27 104.78,88.9 93.34,88.9 92.71,89.53 v92.71,92.08
N$339
  Top 0.305: R4.1 269.24,109.22 SW7.1
N$342  (via drill 0.6)
  Top 0.305: P8.9 26.67,111.44 30.48,115.25 30.48,121.28 34.92,125.73 v34.92,130.18
  Bottom 0.305: IC1.20 66.67,130.81 65.41,129.54 62.23,129.54 61.91,129.86 55.56,129.86 55.24,129.54 36.2,129.54 35.56,130.18 v34.92,130.18
N$343
  Top 0.305: IC31.3 RN23.3 158.75,133.99 160.02,135.25 160.02,140.34 158.75,141.6 IC30.4 | SV12.2 SV11.2
  Bottom 0.305: IC31.3 158.75,127 156.84,125.09 149.22,125.09 148.59,125.73 144.15,125.73 143.51,126.36 SV12.2
N$344
  Top 0.305: IC31.4 RN23.4 161.29,133.99 162.56,135.25 162.56,140.34 163.83,141.6 IC30.6 | SV12.3 SV11.3
  Bottom 0.305: IC31.4 161.29,127 159.38,125.09 158.75,124.46 148.59,124.46 147.96,125.09 141.6,125.09 140.97,125.73 SV12.3
N$345
  Top 0.305: IC31.5 RN23.5 163.83,133.99 165.1,135.25 165.1,137.79 168.91,141.6 IC30.8 | SV11.4 SV12.4
  Bottom 0.305: IC31.5 163.83,128.91 163.19,129.54 149.22,129.54 147.96,128.27 139.7,128.27 SV11.4
N$346
  Top 0.305: IC31.6 RN23.6 | SV12.5 SV11.5
  Bottom 0.305: RN23.6 167.64,130.81 169.54,130.81 170.18,130.18 174.62,130.18 175.26,130.81 175.26,134.62 IC30.11 | IC31.6 166.37,129.54 165.74,130.18 149.54,130.18 148.27,131.44 136.53,131.44 135.89,130.81 SV11.5
N$347
  Top 0.305: IC31.7 RN23.7 IC30.13 | SV11.6 SV12.6
  Bottom 0.305: IC31.7 168.91,129.54 168.28,130.18 166.69,130.18 166.05,130.81 149.86,130.81 148.59,132.08 133.99,132.08 133.35,131.44 SV11.6
N$348  (via drill 0.6)
  Top 0.305: IC31.8 RN23.8 | SV12.7 SV11.7 v130.81,135.89
  Bottom 0.305: RN23.8 171.45,132.72 170.18,133.99 165.74,133.99 IC30.15 163.83,137.16 163.19,137.79 144.46,137.79 141.29,134.62 132.08,134.62 v130.81,135.89
N$350  (via drill 0.6)
  Top 0.305: v212.41,110.49 212.41,110.81 212.72,111.12 212.72,114.94 211.46,116.2 211.46,120.65 v212.09,121.28 | v87.63,135.89 v87.63,129.54
  Bottom 0.305: IC23.3 51.44,138.43 52.39,137.48 62.55,137.48 62.87,137.16 81.92,137.16 83.19,135.89 v87.63,135.89 | SW7.2 264.16,111.76 254.63,111.76 250.19,116.2 250.19,116.84 247.65,119.38 220.34,119.38 213.36,112.39 213.36,111.44 v212.41,110.49 | v212.09,121.28 210.19,119.38 179.71,119.38 179.07,120.02 179.07,122.56 177.8,123.83 147.96,123.83 147.32,124.46 116.2,124.46 115.57,125.09 88.27,125.09 87.63,125.73 v87.63,129.54
N$356  (via drill 0.6)
  Top 0.305: IC31.9 RN23.9 | SV12.8 SV11.8 v128.27,134.62
  Bottom 0.305: RN23.9 172.72,130.81 170.81,130.81 170.18,131.44 170.18,132.72 169.54,133.35 163.83,133.35 162.56,134.62 162.56,136.53 161.93,137.16 160.02,137.16 IC30.17 157.48,137.16 144.78,137.16 141.6,133.99 128.91,133.99 v128.27,134.62
N$357
  Top 0.305: IC31.2 RN23.2 156.21,133.99 154.94,135.25 154.94,140.97 153.67,142.24 IC30.2 | SV11.1 SV12.1
  Bottom 0.305: IC31.2 156.21,127.64 155.57,127 SV12.1
N$358
  Bottom 0.305: IC35.15 175.9,40.64 177.16,41.91 180.34,41.91 181.61,40.64 193.04,40.64 194.31,41.91 219.71,41.91 220.34,41.27 232.41,41.27 233.04,41.27 251.46,41.27 252.73,40.01 IC22.16
N$359  (via drill 0.6)
  Top 0.305: v221.62,42.55 v221.62,39.37
  Bottom 0.305: IC35.13 175.26,35.56 176.53,36.83 180.97,36.83 182.25,38.1 193.04,38.1 194.31,39.37 v221.62,39.37 | IC22.15 255.27,40.64 254,41.91 222.25,41.91 v221.62,42.55
N$360
  Bottom 0.305: IC35.11 173.99,30.48 175.26,31.75 213.36,31.75 216.53,34.92 226.06,34.92 228.92,37.78 261.62,37.78 262.89,39.05 IC22.12
N$361  (via drill 0.6)
  Top 0.305: v224.79,36.2 v224.79,45.09
  Bottom 0.305: IC35.8 193.04,35.56 194.31,36.83 224.16,36.83 v224.79,36.2 | IC22.9 262.89,45.72 261.62,44.45 243.52,44.45 242.89,45.09 225.43,45.09 v224.79,45.09
N$362
  Route2 0.305: IC35.6 193.04,40.64 194.31,41.91 220.34,41.91 220.98,41.27 251.46,41.27 255.27,45.09 IC22.6
N$363
  Bottom 0.305: IC35.4 193.04,45.72 194.31,46.99 214.63,46.99 215.9,48.26 243.21,48.26 243.84,47.62 243.84,46.35 244.47,45.72 252.09,45.72 252.73,46.35 IC22.5
N$364
  Bottom 0.305: IC22.2 245.11,47.62 243.84,48.9 211.46,48.9 210.82,49.53 193.68,49.53 192.41,48.26 181.61,48.26 IC35.2
N$365
  Top 0.305: RN6.9 147.32,121.92 147.32,116.84 U10.K0
N$366
  Top 0.305: RN6.8 143.51,122.56 144.78,121.28 144.78,117.47 143.51,116.2 U10.K1
N$367
  Top 0.305: RN6.7 140.97,122.56 142.24,121.28 142.24,117.47 140.97,116.2 U10.K2
N$368
  Top 0.305: RN6.6 138.43,121.92 139.7,120.65 139.7,117.47 138.43,116.2 U10.K3
N$369
  Top 0.305: RN6.5 135.89,121.92 137.16,120.65 137.16,117.47 135.89,116.2 U10.K4
N$370
  Top 0.305: RN6.4 133.35,121.92 134.62,120.65 134.62,117.47 133.35,116.2 U10.K5
N$371
  Top 0.305: RN6.3 130.81,121.92 132.08,120.65 132.08,117.47 130.81,116.2 U10.K6
N$372
  Top 0.305: RN6.2 128.27,121.92 129.54,120.65 129.54,117.47 128.27,116.2 U10.K7
N$373  (via drill 0.6)
  Top 0.305: U10.A3 138.43,120.65 137.16,121.92 137.16,133.99 v139.06,135.89
  Bottom 0.305: IC30.12 171.45,136.53 168.91,139.06 142.24,139.06 v139.06,135.89
N$374  (via drill 0.6)
  Top 0.305: U10.A2 140.97,120.65 139.7,121.92 139.7,134.62 v140.97,135.89
  Bottom 0.305: IC30.14 166.37,137.79 165.74,138.43 143.51,138.43 v140.97,135.89
N$375  (via drill 0.6)
  Top 0.305: U10.A1 143.51,121.28 142.24,122.56 142.24,130.49 v144.78,133.03
  Bottom 0.305: IC30.16 161.29,134.62 160.66,133.99 151.45,133.99 150.5,133.03 v144.78,133.03
N$376  (via drill 0.6)
  Top 0.305: U10.A0 146.05,121.28 144.78,122.56 144.78,130.81 147.32,133.35 v147.32,133.99
  Bottom 0.305: IC30.18 154.94,134.62 150.5,134.62 149.86,133.99 v147.32,133.99
N$377  (via drill 0.6)
  Top 0.305: U10.A4 135.89,120.65 134.62,121.92 v134.62,135.89
  Bottom 0.305: IC30.9 171.45,142.24 168.91,139.7 140.97,139.7 137.16,135.89 v134.62,135.89
N$378  (via drill 0.6)
  Top 0.305: U10.A5 133.35,120.65 132.08,121.92 132.08,135.25 v132.72,135.89
  Bottom 0.305: IC30.7 166.37,142.24 164.47,140.34 140.34,140.34 137.16,137.16 133.99,137.16 v132.72,135.89
N$379  (via drill 0.6)
  Top 0.305: U10.A6 130.81,120.65 129.54,121.92 v129.54,135.89
  Bottom 0.305: IC30.5 161.29,142.88 159.38,140.97 139.7,140.97 137.16,138.43 130.81,138.43 129.54,137.16 v129.54,135.89
N$380  (via drill 0.6)
  Top 0.305: IC30.3 156.21,138.43 157.48,137.16 v157.48,122.56
  Bottom 0.305: v157.48,122.56 157.48,119.38 156.84,118.75 147.32,118.75 146.69,119.38 128.91,119.38 128.27,118.75 U10.A7
N$381
  Bottom 1.422: S1.8 S1.7 S1.6 S1.5 S1.4 S1.3 S1.2 S1.1 199.39,140.97 203.2,137.16 R39.1
N$382
  Top 0.305: S1.9 RN24.2 SV2.8 SV7.8
N$383
  Top 0.305: S1.10 RN24.3 SV2.7 SV7.7
N$384
  Top 0.305: S1.11 RN24.4 SV2.6 SV7.6
N$385
  Top 0.305: S1.12 RN24.5 SV2.5 SV7.5
N$386
  Top 0.305: SV10.5 SV8.5 RN8.6 97.79,136.53 98.42,137.16 113.67,137.16 114.3,136.53 114.3,107.95 118.11,104.14 118.11,90.17 119.38,88.9 119.38,85.09 123.19,81.28 IC28.11
  Route2 0.305: IC29.6 74.93,77.47 76.2,78.74 76.2,80.64 77.47,81.92 122.56,81.92 123.19,81.28 IC28.11
N$387
  Top 0.305: S1.14 RN24.7 SV2.3 SV7.3
N$388
  Top 0.305: S1.15 RN24.8 SV2.2 SV7.2
N$389
  Top 1.422: R38.1 206.38,5.08 205.74,4.45 SW17.1
N$397
  Top 0.305: SV3.8 RN26.2
  Bottom 0.305: IC37.17 181.61,93.98 178.44,90.81 177.16,90.81 176.53,90.17 SV3.8
N$398
  Top 0.305: RN7.9 U11.K0
N$399
  Top 0.305: RN7.8 U11.K1
N$400
  Top 0.305: RN7.7 U11.K2
N$401
  Top 0.305: RN7.6 U11.K3
N$402
  Top 0.305: RN7.5 U11.K4
N$403
  Top 0.305: RN7.4 U11.K5
N$404
  Top 0.305: RN7.3 U11.K6
N$405
  Top 0.305: RN7.2 U11.K7
N$406
  Top 0.305: SV3.7 RN26.3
